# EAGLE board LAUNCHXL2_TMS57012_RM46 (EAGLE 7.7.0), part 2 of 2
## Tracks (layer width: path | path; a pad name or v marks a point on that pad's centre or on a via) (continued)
HERCULES_LIN1_TXD  (via drill 0.38 pad 0.69) (continued)
  Bottom 0.152: v58.09,41.15 58.09,58.61 57.65,59.04 51.78,59.04 51.48,59.35 51.48,63.18 51.17,63.48 48.28,63.48 47.98,63.79 47.98,66.09 47.68,66.4 25.12,66.4 J10.9 | v93.2,8.9 93.13,4.67 93.43,4.37 94.94,4.37 95.25,4.67 J6.4 | v85.56,28.32 85.56,28.11 85.27,27.81 85.26,23.32 84.95,23.01 78.35,23.01 78.04,22.71 78.08,14.22 76.76,12.75 76.45,12.39 v76.47,9.45 | v69.54,41.15 90.49,41.15 v90.75,40.9 91.21,40.43 91.21,40.39 v91.13,31.5
HERCULES_MR_PB  (via drill 0.38 pad 0.56, 0.38 pad 0.69)
  Top 0.152: S1.4 125.89,44.35 v119.43,44.35 117.94,44.35 S1.3 | v51.99,45.06 U7.40 | v119.43,49.92 120.14,49.92 120.14,51 U2.3 117.22,51 116.92,51.31 116.92,54.23 117.22,54.53 124.26,54.53 124.26,57.2 113.62,57.2 111.67,55.24 | 111.67,55.24 | 111.67,55.24 109.55,55.24 109.25,55.55 109.25,61.2 108.94,61.51 v95.87,61.51 | v79.48,51.61 52.56,51.46 v51.99,52.03 51.91,52.12 44.12,52.12 43.97,52.27 42.44,52.27 42.29,52.12 25.15,52.12 24.46,52.81 v17.68,52.81 | J1.15 4.83,53.21 4.65,53.03 v4.57,53.03 | v79.48,61.42 79.53,61.47 81.28,61.47 81.53,61.59 81.55,61.58 v92.56,61.58
  Bottom 0.152: v51.99,52.03 v51.99,45.06 | v119.43,44.35 v119.43,49.92 | v79.48,51.61 v79.48,61.42 | v4.57,53.03 4.57,52.5 7.01,50.06 15.32,50.06 16.38,51.36 17.53,52.81 v17.68,52.81 | v92.56,61.58 92.63,61.51 v95.87,61.51
HERCULES_NRST  (via drill 0.38 pad 0.69)
  Top 0.152: v56.16,57.81 55.52,57.78 53.47,57.78 53.09,58.04 34.92,58.04 34.59,57.81 34.29,57.51 J5.5 | v93.28,58.95 93.28,60.67 93.07,60.88 92.05,60.88 91.85,61.09 81.92,61.09 81.53,60.71 75.82,60.71 75.42,60.97 v74.73,61.54 | v57.51,62.91 v50.62,62.91 | v121.21,49.28 R10.1 | v54.93,35.26 U7.25 | v111.21,62.08 114.46,62.08 116.47,63.7 122.38,63.7 122.97,63.12 v123.29,63.12 | v97.79,62.08 v109.66,62.08 | J9.5 98.78,55.52 98.78,52.12 98.39,51.73 v92.71,51.73 | 124.39,33.31 | 124.39,33.31 S2.4 | S2.4 | 124.39,33.31 v123.05,33.31 S2.3
  Top 0.203: 99.59,47.92 99.16,47.57 98.88,47.57 98.81,47.3 98.81,46.79 | 98.81,46.79 98.81,45.34 | 98.81,46.79 v98.59,46.79
  Top 0.254: C3.1 99.59,47.92 | 98.81,45.34 U1.116
  Bottom 0.152: v93.28,58.95 96.24,58.95 96.55,58.65 96.55,56.52 J9.5 v97.79,62.08 | J10.22 57.15,63.82 v57.51,62.91 57.51,62.89 58.67,61.72 74.55,61.72 v74.73,61.54 | v123.05,33.31 123.05,45.25 121.21,47.09 v121.21,49.28 123.29,51.36 123.29,58.52 123.6,58.83 123.6,62.81 v123.29,63.12 | v50.62,62.91 50.62,58.91 50.93,58.61 55.28,58.61 v56.16,57.81 56.24,57.3 56.77,56.77 56.77,56.24 57,56.01 57,49.38 56.77,49.15 56.77,47.7 56.92,47.55 56.92,37.25 v54.93,35.26 | v109.66,62.08 v111.21,62.08 | v92.71,51.73 92.71,48.72 93.12,48.31 97.07,48.31 v98.59,46.79
HERCULES_NTRST  (via drill 0.38 pad 0.56, 0.38 pad 0.69)
  Top 0.152: v46.38,25.52 U7.107 | v68.82,48.88 68.81,48.9 68.2,48.9 68.07,48.77 52.32,48.77 51.96,49.14 v46.43,49.14 45.24,49.95 26.18,49.95 25.76,49.53 22.71,49.53 v22.55,49.76 | J1.2 v14.94,62.1 | v90.06,38.65 98.42,38.65 101.73,42.04 101.73,43.81 102.3,44.39 U1.109
  Bottom 0.152: v68.82,48.88 68.82,40.88 69.12,40.58 89.68,40.58 89.98,40.27 v90.06,38.65 | v46.43,49.14 45.09,47.67 45.09,40.46 46.38,39.17 v46.38,25.52 | v22.55,49.76 22.55,52.65 19.89,55.32 17.98,55.32 15.7,57.61 15.7,61.8 15.39,62.1 v14.94,62.1
HERCULES_RTCK  (via drill 0.38 pad 0.56, 0.38 pad 0.69)
  Top 0.152: v99.14,41.84 99.63,41.92 100.39,42.68 100.39,43.99 100.32,44.06 U1.113 | v86.48,38.17 87.1,37.87 87.4,37.57 v98.15,37.56 | v45.66,32.39 53.45,32.39 53.76,32.69 53.76,38.09 54.06,38.4 v67,38.4 | v46.25,22.87 46.49,22.87 46.79,23.16 U7.108 | J1.9 4.67,57.02 v4.72,56.92
  Bottom 0.152: v98.15,37.56 99.19,38.48 v99.14,41.84 | v67,38.4 74.61,38.4 74.85,38.16 81.7,38.16 83.46,39.92 86.19,39.92 86.33,39.78 86.33,38.79 86.49,38.71 86.49,38.56 v86.48,38.17 | v46.25,22.87 45.66,24.08 v45.66,32.39 44.56,31.3 44.56,29.55 44.26,29.25 41.66,29.25 41.27,29.63 41.27,40.13 41.02,40.39 41.02,41.4 41.27,41.66 41.27,45.09 40.64,45.72 36.2,45.72 35.69,46.23 21.19,46.19 20.88,46.49 20.88,53.73 20.04,54.57 15.3,54.57 15.01,55.02 15.01,56.08 14.71,56.39 5.11,56.39 v4.72,56.92
HERCULES_TCK  (via drill 0.38 pad 0.56, 0.38 pad 0.69)
  Top 0.152: v79.46,46.93 78.96,47.43 61.69,47.43 61.4,47.13 54.3,47.13 54,46.83 U7.35 | U1.112 100.8,42.35 99.47,41.02 98.65,41.02 98.15,41.67 v97.46,41.67 | v16,52.96 16.77,52.27 16.76,52.26 16.76,51.51 17.14,51.13 19.2,51.13 19.66,51.59 24.16,51.59 24.46,51.28 42.37,51.28 42.6,51.05 43.81,51.05 44.2,51.44 51.82,51.44 52.32,50.93 57.15,50.93 57.4,50.8 78.79,50.85 79.15,50.62 v79.46,50.09 | J1.11 7.02,55.7 4.57,55.7 v4.12,55.55
  Bottom 0.152: v97.46,41.67 97.46,42.72 96.77,43.41 96.77,44.45 95.89,45.34 79.99,45.34 79.46,45.88 v79.46,46.93 v79.46,50.09 | v4.12,55.55 8.53,55.55 9.98,54.1 14.55,54.1 v16,52.96
HERCULES_TDI  (via drill 0.38 pad 0.56, 0.38 pad 0.69)
  Top 0.152: v100.75,46.55 101.82,46.55 U1.110 | v52.59,42.66 52.78,42.47 | 52.78,42.47 | 52.78,42.47 U7.38 | 6.92,60.88 J1.3 6.94,60.81 5.03,60.81 2.59,58.37 2.59,50.9 4.19,49.3 14.33,49.3 15.28,50.25 21.68,50.25 22.1,50.67 23.32,50.67 23.7,50.29 49.3,50.29 49.76,49.84 52.35,49.84 v52.59,49.59 52.65,49.53 66.6,49.53 66.98,49.91 70.03,49.91 70.64,49.3 76.66,49.3 77.11,48.84 79.86,48.84 80.68,49.75 v80.95,49.75
  Bottom 0.152: v52.59,49.59 v52.59,42.66 | v100.75,46.55 100.69,46.18 81.99,46.18 80.47,47.7 80.47,48.77 80.92,49.23 80.92,49.72 v80.95,49.75
HERCULES_TDO  (via drill 0.38 pad 0.56, 0.38 pad 0.69)
  Top 0.152: v53.19,38.19 U7.37 | J1.7 4.04,58.29 v3.73,58.22 | v14.71,59.44 15.54,59.44 19.43,55.55 21.49,55.55 21.79,55.24 32.31,55.24 32.61,55.02 35.74,55.02 36.12,55.32 45.11,55.32 45.41,55.02 47.93,55.02 48.08,54.86 53.09,54.86 v53.03,54.89 | U1.111 101.35,45.28 101.35,44.32 101.22,44.07 101.22,42.16 99.43,40.38 98.2,39.27 88.77,39.27 87.55,40.39 84.67,40.38 84.37,40.81 84.37,44.14 83.81,45.46 55.21,45.46 55.02,45.26 55.02,44.61 v54.98,44.58
  Bottom 0.152: v53.19,38.19 53.11,41.83 53.26,42.14 53.26,42.67 53.19,43.05 53.19,45.42 | 53.19,45.42 53.11,48.92 53.34,49.23 53.34,49.84 53.11,50.14 v53.03,54.89 | v3.73,58.22 13.49,58.22 v14.71,59.44 | 53.19,45.42 54.15,45.42 v54.98,44.58
HERCULES_TMS  (via drill 0.38 pad 0.56, 0.38 pad 0.69)
  Top 0.152: v99.08,58.32 99.08,52.77 99.59,52.27 104.39,52.27 104.78,51.89 v104.78,51.56 | v54.57,54.89 55.12,54.86 | 55.12,54.86 54.99,54.86 | 55.12,54.86 74.42,54.86 74.55,54.99 75.31,54.99 75.44,54.86 80.26,54.86 80.77,54.48 84.71,54.48 85.18,54.59 85.41,55.12 85.41,55.99 v84.75,56.81 | v54.57,47.71 53.9,47.71 53.59,47.4 U7.36 | J1.1 v4.88,62.1 | v15.01,51.82 16.31,50.67 19.66,50.67 20.19,51.21 23.77,51.21 24.16,50.83 41.45,50.83 41.6,50.67 44.65,50.67 45.03,51.05 51.13,51.05 51.66,50.52 54.37,50.52 v54.5,50.32 | v104.78,48.22 104.78,44.58 104.27,44.07 104.27,43.35 U1.108
  Bottom 0.152: v84.75,56.81 84.75,63.93 85.05,64.24 88.16,64.24 89.59,62.73 98.78,62.73 99.08,62.34 v99.08,58.32 | v54.57,47.71 v54.5,50.32 v54.57,54.89 | v15.01,51.82 11.96,51.82 11.05,52.73 10.06,52.73 8.15,54.63 3.89,54.63 2.82,55.7 2.82,58.6 4.57,60.35 4.57,61.8 v4.88,62.1 | v104.78,48.22 104.78,49 105.16,49.38 105.16,49.99 104.85,50.29 104.85,51.48 v104.78,51.56
IRSTN  (via drill 0.38 pad 0.69)
  Top 0.152: R39.2 v38.12,34.41
  Top 0.178: R39.2 38.61,35.36 39.4,36.05 U7.70 | J12.10 v13.36,25.91
  Bottom 0.152: v38.12,34.41 39.5,34.42 40.51,33.53 40.51,28.07 39.88,27.43 37.72,25.4 37.72,25.38 37.34,25.15 35.05,25.15 34.82,25.38 34.59,25.38 27.18,25.4 26.04,25.02 20.07,25.02 19.18,25.91 v13.36,25.91
ITCK  (via drill 0.38 pad 0.69)
  Top 0.152: U7.100 43.59,25.65 44.15,26.21 v44.3,26.21 | 26.54,23.62 15.62,23.62 15.24,24 15.24,25.78
  Top 0.178: J12.4 14.73,29.72 15.24,29.21 15.24,25.78 | 26.54,23.62 29.59,19.56 38.73,19.56 v41.35,22.17
  Bottom 0.178: v41.35,22.17 41.35,23.27 v44.3,26.21
ITDI
  Top 0.152: 25.78,22.48 15.49,22.48 14.35,23.75 14.35,25.4
  Top 0.178: U7.98 42.8,21.84 39.5,18.41 28.7,18.41 25.78,22.48 | 14.35,25.4 14.35,26.8 14.1,27.05 11.3,27.05 J12.8
ITDO
  Top 0.152: U7.97 | 14.86,25.53 14.86,23.75 15.49,23.11 26.04,23.11
  Top 0.178: 42.37,24.21 U7.97 42.42,24.21 42.39,23.77 42.39,23.36 42.37,23.33 42.29,23.24 42.29,22.1 41.53,21.34 41.4,21.34 39.12,19.05 29.08,19.05 26.04,23.11 | J12.6 14.22,28.45 14.86,27.81 14.86,25.53
ITMS
  Top 0.152: 41.48,23.82 41.48,23.42 | 15.75,26.04 15.75,24.13 15.88,24 27.05,24
  Top 0.178: 41.48,23.82 41.48,24.84 41.99,25.35 43.08,25.35 43.18,25.25 U7.99 | J12.2 14.22,30.99 15.75,29.46 15.75,26.04 | 27.05,24 30.1,20.07 38.25,20.07 41.48,23.42
KGND
  Top 0.152: 82.8,34.39 U1.19
  Top 0.178: C2.2 C1.2 80.61,34.39 81.45,34.39 81.63,34.34 82.37,34.34 82.8,34.39
MIBSPI1CLK  (via drill 0.38 pad 0.69)
  Top 0.152: J6.7 101.6,12.06 101.6,14.86 101.91,15.16 102.37,15.16 102.67,15.47 102.67,27.75 102.37,28.05 100.28,28.05 99.98,28.36 v99.98,33.7 100.7,34.42 100.7,36.56 101,36.86 U1.95
  Bottom 0.152: v99.98,33.7 94.8,33.7 94.5,34.01 94.5,44.07 93.81,44.89 83.69,44.83 79.5,44.83 79.45,44.89 79.02,45.27 78.72,45.57 78.72,63.64 79.02,63.94 81.09,63.94 J10.32
MIBSPI1NCS_0/MIBSPI1SOMI_1/MII_TXD_2/ECAP6  (via drill 0.38 pad 0.56)
  Top 0.152: J9.3 92.71,59.77 92.28,60.2 91.82,60.2 91.31,60.71 82.42,60.71 81.92,60.2 71.37,60.2 68.96,62.61 68.96,63.75 J10.26 | U1.105 103.07,41.84 102.74,42.16 102.74,43.05 102.87,43.18 102.87,46.94 102.41,47.4 102.11,47.4 v101.58,47.85
  Bottom 0.152: J9.3 93.73,55.5 93.73,52.12 94.64,51.21 94.64,50.75 94.49,50.6 94.49,50.14 94.94,49.68 99.97,49.68 v101.58,47.85
MIBSPI1NCS_1/N2HET1_17/MII_COL/EQEP1S  (via drill 0.38 pad 0.69)
  Top 0.152: v90.73,47.73 90.89,47.54 91.81,46.61 U1.130 | v82.82,63.5 76.63,63.5 76.2,64.06 76.2,66.09 75.89,66.4 30.77,66.4 J10.11 | v82.82,60.1 90.51,60.1 v90.93,59.52 | v95,59.52 105.11,59.52 105.41,59.22 J9.8
  Bottom 0.152: v82.82,63.5 v82.82,60.1 82.83,58.22 82.37,57.76 82.37,56.39 82.82,55.94 82.82,55.64 82.83,55.63 82.82,48.77 83.12,48.34 84.75,48.34 84.96,48.13 85.98,48.13 86.23,48.39 90.19,48.39 v90.73,47.73 | v95,59.52 v90.93,59.52
MIBSPI1NCS_2/N2HET1_19/MDIO  (via drill 0.38 pad 0.69)
  Top 0.152: v86.33,25.15 86.33,25.87 86.49,26.04 87.16,26.04 v87.55,26.34 | v113.6,52.68 107.01,52.68 106.7,52.98 106.7,55.27 J9.9 | v86.33,25.15 | v86.33,25.15 U1.40
  Bottom 0.152: v86.33,25.15 86.33,22.44 86.02,22.14 81.31,22.14 81,21.83 81,2.9 J11.31 | v113.6,52.68 113.6,29.91 113.3,29.6 89.44,29.6 89.13,29.91 89.13,39.19 88.96,39.37 87.65,39.37 87.47,39.19 v87.55,26.34
MIBSPI1NENA/N2HET1_23/MII_RXD_2/ECAP4  (via drill 0.38 pad 0.69)
  Top 0.152: J8.4 93.85,55.37 v93.85,60.67 | v85.32,63.67 84.81,64.18 81.24,64.18 J10.31 | v100.13,37.28 103.73,37.28 103.8,37.34 U1.96
  Bottom 0.152: v85.32,63.67 85.32,60.97 85.62,60.67 v93.85,60.67 | J8.4 97.1,52.12 98.75,52.12 99.52,51.36 103.02,51.36 103.17,51.21 103.17,47.7 103.02,47.55 103.02,45.11 102.56,44.64 100.7,44.64 100.39,44.34 100.39,37.55 v100.13,37.28
MIBSPI1SIMO  (via drill 0.38 pad 0.69)
  Top 0.152: v110.5,38.47 110.5,36.15 110.2,35.84 U1.93 | J9.6 101.6,55.24 106.1,55.24 106.4,54.94 106.4,51.44 106.88,50.98 v110.48,50.98
  Bottom 0.152: J9.6 100.33,62.65 99.8,63.11 92.62,63.11 J10.35 | v110.48,50.98 110.48,50.93 v110.5,38.47
MIBSPI1SOMI  (via drill 0.38 pad 0.69)
  Top 0.152: v106.04,37.52 106.04,36.66 105.73,36.35 U1.94
  Bottom 0.152: J10.33 86.08,66.4 101.4,66.4 101.7,66.09 101.7,57.68 J9.7 101.7,55.35 101.7,53.56 102.11,52.96 105.46,52.96 105.77,52.65 105.77,52.19 105.77,52.18 105.77,43.69 106.08,43.38 106.28,43.38 106.58,43.08 106.58,42.52 105.47,41.4 105.47,38.09 v106.04,37.52
MIBSPI3CLK/AWM_EXT_SEL_1/EQEP1A  (via drill 0.38 pad 0.69)
  Top 0.152: v87.2,15.53 87.63,15.49 92.08,15.49 92.78,16.32 92.8,16.9 U1.53 | v87.24,6.77 v39.37,6.77 | v87.24,4.21 v97.79,4.21
  Bottom 0.152: 86.45,7.55 v87.24,6.77 v87.24,4.21 | 86.45,7.55 | 86.45,7.55 86.45,14.94 v87.2,15.53 | v39.37,6.77 J2.7 | v97.79,4.21 J11.38
MIBSPI3NCS_0/AD2EVT/GIOB_2/EQEP1I  (via drill 0.38 pad 0.69)
  Top 0.152: v93.14,25.26 93.82,25.26 U1.55 | J6.5 97.79,9.63 98.09,9.32 111.73,9.32 112.03,9.63 112.03,26.77 v112.09,26.9 112.62,26.83 113.54,25.91 | 123.12,23.15 S3.3 113.76,23.15 113.54,23.37 113.54,25.91 | 123.12,23.15 | 123.12,23.15 S3.4 | S3.4 | 113.54,25.91 113.79,26.16 R13.1
  Bottom 0.152: J6.5 97.79,5.84 98.09,5.54 102.56,5.54 102.87,5.23 J11.40 | v112.09,26.9 112.03,26.89 100.13,26.82 99.9,27.28 97.69,27.28 96.32,28.65 94.72,28.65 94.34,28.04 94.34,27.77 93.14,26.58 v93.14,25.26
MIBSPI3NCS_1/N2HET1_25/MDCLK  (via drill 0.38 pad 0.69)
  Top 0.152: v64.99,58.08 64.99,59.49 63.92,60.3 38.89,60.3 v37.53,61.4 | v37.53,61.4 | v77.47,21.12 69.56,21.12 69.25,21.43 69.25,26.79 70.97,28.5 70.97,34.11 v72.95,35.94 | v84.69,25.42 84.83,25.28 U1.37
  Bottom 0.152: v37.53,61.4 33.35,61.4 33.05,61.1 33.05,52.98 32.74,52.68 30.95,52.68 30.64,52.98 30.64,55.08 J5.3 | v72.95,35.94 65.29,35.94 64.99,36.25 v64.99,58.08 | v84.69,25.42 82.82,23.55 77.78,23.55 77.47,23.25 v77.47,21.12 77.47,14.43 75.89,12.8 75.69,12.6 75.74,4.95 75.44,4.65 75.44,3.73 75.69,3.48 75.69,3.15 J11.30
MIBSPI3NCS_2/I2C_SDA/N2HET1_27/NTZ2  (via drill 0.38 pad 0.69)
  Top 0.152: v62.46,42.68 63.36,43.2 69.85,43.18 70.1,43.18 | 78.42,41.84 78.49,41.84 | 78.49,41.84 U1.4 | v56.02,50.17 v62.46,50.17 | v22.23,15.24 24.26,15.24 24.77,15.75 25.43,16.42 25.73,16.73 66.63,16.73 66.93,17.03 66.93,32.69 70.19,35.87 70.18,37.87 70.79,38.56 70.79,42.22 70.11,42.73 70.1,43.18 | 70.1,43.18 77.11,43.18 78.3,41.86 78.46,41.86 78.49,41.84
  Bottom 0.152: v62.46,50.17 v62.46,42.68 | v56.02,50.17 56.02,50.2 55.4,50.83 55.41,56.74 54.62,57.53 48.64,57.53 48.26,57.91 44.07,57.91 42.67,56.52 J5.8 | v22.23,15.24 21.72,14.61 21.72,10.79 24,8.64 24,2.92 J11.9
MIBSPI3NCS_3/I2C_SCL/N2HET1_29/NTZ1  (via drill 0.38 pad 0.69)
  Top 0.152: v59.62,43.76 77.45,43.76 78.86,42.35 U1.3 | J5.9 45.7,55.42 52.1,55.42 52.37,55.54 v59.62,55.54 | v43.18,51.69 24.74,51.69 24.31,52.12 19.18,52.12 v18.82,51.84
  Bottom 0.152: J5.9 43.18,55.24 v43.18,51.69 | J11.8 20.4,0.71 18.09,0.71 17.78,1.02 17.78,2.34 14.48,5.64 14.48,7.16 13.87,7.77 13.44,7.77 13.36,7.86 3.7,7.86 3.4,8.16 3.4,27.48 4.04,28.12 4.19,28.32 4.19,31.11 3.3,32.13 1.91,33.27 1.91,48.9 2.79,49.78 5.97,49.78 6.22,49.53 16.51,49.53 v18.82,51.84 | v59.62,55.54 v59.62,43.76
MIBSPI3NENA/MIBSPI3NCS_5/N2HET1_31/EQEP1B  (via drill 0.38 pad 0.69)
  Top 0.152: v99.13,17.95 98.86,17.68 97.61,17.68 97.54,17.6 93.73,17.6 93.62,17.72 93.31,18.02 U1.54 | v100.33,6.66 v100.33,4.97
  Bottom 0.152: J6.8 105.41,6.97 105.11,6.66 v100.33,6.66 100.33,7.27 99.13,8.47 v99.13,17.95 | v100.33,4.97 J11.39
MIBSPI3SIMO/AWM_EXT_SEL_0/ECAP3  (via drill 0.38 pad 0.69)
  Top 0.152: v89.19,8.88 v60.93,8.88 | v60.93,23.6 55.44,23.6 55.13,23.9 55.13,26.14 51.43,29.84 v43.24,29.84 | v89.19,16.41 92.02,16.41 92.32,16.84 U1.52
  Bottom 0.152: J11.37 94.06,0.71 91.75,0.71 91.44,1.02 91.44,4.07 89.19,6.32 v89.19,8.88 89.18,8.9 89.18,15.76 v89.19,16.41 | v43.24,29.84 43.24,49.16 42.94,49.47 35.89,49.47 35.59,49.77 35.59,55.27 J5.6 | v60.93,23.6 v60.93,8.88
MIBSPI3SOMI/AWM_EXT_ENA/ECAP2  (via drill 0.38 pad 0.69)
  Top 0.152: v56.17,40.27 v67.79,40.27 | v91.47,17.72 91.94,18.19 91.94,22.55 91.81,22.67 U1.51
  Bottom 0.152: v91.47,17.72 | v91.47,17.72 91.47,9.13 92.71,7.89 J11.36 | v91.47,17.72 89.22,17.72 88.93,18.01 | 88.93,18.01 | 88.93,18.01 81.85,18.01 81.55,18.32 81.55,21.26 81.85,21.57 86.59,21.57 86.94,21.92 86.94,25.38 86.87,34.29 86.87,35.36 87.17,35.59 87.1,39.85 86.59,40.27 v67.79,40.27 | v56.17,40.27 56.16,49.38 56.17,49.38 56.17,49.46 56.62,49.91 56.62,50.67 56.16,51.13 56.17,56.67 54.67,58.17 49.66,58.17 49.28,58.55 41.4,58.55 J5.7
MIBSPI5CLK/MII_TXEN/RMII_TXEN  (via drill 0.38 pad 0.69)
  Top 0.152: J8.10 109.25,53.98 108.94,54.28 108.94,60.36 108.64,60.67 95.03,60.67 94.73,60.97 94.73,62.19 94.42,62.5 75.51,62.56 75.36,62.71 74.14,62.71 73.93,62.5 72.76,62.5 J10.27 | v108.83,38.8 106.42,38.8 105.87,39.35 U1.100
  Bottom 0.152: J8.10 110.49,52.18 108.83,50.52 | 108.83,50.52 | 108.83,50.52 v108.83,38.8
MIBSPI5NCS_0/EPWM4A  (via drill 0.38 pad 0.69)
  Top 0.152: U1.32 82.91,27.81 84.05,27.81 84.12,27.74 84.12,27.19 v84.15,27.16
  Bottom 0.152: v84.15,27.16 81.35,25.12 78.39,25.12 78.12,25.39 67.61,25.39 67.31,25.08 J11.26
MIBSPI5NENA/MII_RXD_3/MIBSPI5SOMI_1/ECAP5  (via drill 0.38 pad 0.69)
  Top 0.152: v87.06,63.59 86.33,64.01 86.33,66.06 86.07,66.4 78.46,66.4 J10.30 | J8.5 96.55,55.22 96.55,57.73 v97.12,58.31 | v103.05,37.85 U1.97
  Bottom 0.152: v97.12,58.31 97.12,61.77 96.74,62.23 87.44,62.23 87.06,62.53 v87.06,63.59 | v103.05,37.85 103.33,38.13 103.33,47.09 103.33,47.4 103.48,47.55 103.48,51.51 103.33,51.66 101.35,51.66 100.74,52.27 99.49,52.27 J8.5
MIBSPI5SIMO_0/MII_TXD_1/RMII_TXD_1/MIBSPI5SOMI_2  (via drill 0.38 pad 0.56, 0.38 pad 0.69)
  Top 0.152: v101.38,38.46 102.32,38.46 102.72,38.86 104.09,38.86 U1.99 | J9.4 95.25,57.74 94.42,58.57 94.42,61.81 94.06,62.18 91.75,62.18 91.59,62.03 80.92,62.03 80.77,62.18 78.94,62.18 78.49,61.72 75.74,61.72 75.29,62.26 74.22,62.26 73.98,62.12 71.49,62.12 v70.1,63.5
  Bottom 0.152: J9.4 95.25,55.27 95.56,54.97 98.77,54.97 99.07,54.66 99.07,53.18 99.52,52.73 100.89,52.73 101.35,52.27 103.63,52.27 103.94,51.97 103.94,50.29 103.78,49.99 103.78,47.55 103.94,47.4 103.94,37.58 103.33,36.98 102.6,36.98 101.38,37.43 v101.38,38.46 | v70.1,63.5 71.88,63.5 72.14,63.75 72.14,65.15 J10.28
MIBSPI5SOMI_0/MII_TXD_0/RMII_TXD_0  (via drill 0.38 pad 0.69)
  Top 0.152: J9.10 110.49,62.5 110.12,62.87 95.25,62.87 95,63.12 88.21,63.12 88.01,62.99 84.96,62.99 84.84,63.12 83.44,63.12 83.19,62.87 82.42,62.87 82.3,62.99 75.56,62.99 75.36,63.18 74.93,63.49 J10.29 | U1.98 107.49,38.36 108.66,37.19 109.41,37.19 v109.51,37.29
  Bottom 0.152: J9.10 111.56,55.45 111.56,53.34 111.25,53.03 111.25,50.75 111.1,50.6 111.1,39.47 111.48,39.09 111.48,38.33 110.8,37.64 109.86,37.64 v109.51,37.29
N2HET1_0/SPI4CLK/EPWM2B  (via drill 0.38 pad 0.69)
  Top 0.152: v84.08,31.35 U1.25
  Bottom 0.152: v84.08,31.35 80.24,31.35 78.83,29.93 60.58,29.93 60.27,29.63 60.27,4.66 59.97,4.36 54.52,4.36 J11.20
N2HET1_1/SPI4NENA/N2HET2_8/EQEP2A  (via drill 0.38 pad 0.69)
  Top 0.152: v77.91,58.95 v87.96,58.95 | v93.69,32.34 93.34,32.51 85.17,32.51 v85.09,32.59 84.84,32.34 U1.23 | U1.23
  Bottom 0.152: J11.21 56.41,3.7 61.42,3.7 61.73,4.01 61.73,29.22 62.03,29.53 73.94,29.53 74.94,28.52 79.51,28.52 80.3,29.31 84.34,29.31 84.8,29.62 84.8,31.36 85.09,31.8 v85.09,32.59 | v93.69,32.34 93.69,43.64 93.13,44.45 83.69,44.45 79.63,44.45 79.24,44.45 78.47,45.09 77.91,45.65 v77.91,58.95 | v87.96,58.95 90.17,56.74 J9.2
N2HET1_2/SPI4SIMO/EPWM3A  (via drill 0.38 pad 0.69)
  Top 0.152: v84.08,28.74 83.96,28.86 U1.30
  Bottom 0.152: v84.08,28.74 83.89,28.92 81.09,28.92 80.12,27.95 62.53,27.95 62.23,27.65 J11.24
N2HET1_3/SPI4NCS_0/N2HET2_10/EQEP2B  (via drill 0.38 pad 0.69)
  Top 0.152: v71.12,24.82 77.51,24.82 77.81,25.12 77.81,31.55 78.12,31.86 U1.24
  Bottom 0.152: v71.12,24.82 71.12,1.02 70.81,0.71 58.34,0.71 J11.22
N2HET1_4/EPWM4B  (via drill 0.38 pad 0.69)
  Top 0.152: v69.85,9.45 45.79,9.45 J2.9 | v69.85,23.68 82.54,23.68 82.85,23.98 U1.36
  Bottom 0.152: J11.27 v69.85,9.45 v69.85,23.68
N2HET1_5/SPI4SOMI/N2HET2_12/EPWM3B  (via drill 0.38 pad 0.69)
  Top 0.152: v81.36,28.35 U1.31
  Bottom 0.152: v81.36,28.35 81.36,26.99 81.06,26.68 65.08,26.68 64.77,26.38 J11.25
N2HET1_6/SCIRX/EPWM5A  (via drill 0.38 pad 0.69)
  Top 0.152: J11.33 81.62,5.38 49.48,5.38 49.02,5.89 45.36,5.89 44.86,5.49 33.56,5.49 29.21,9.54 J2.3 | v85.08,17.07 85.08,17.42 85.34,17.68 U1.38
  Bottom 0.152: J11.33 85.09,16.85 v85.08,17.07
N2HET1_7/N2HET2_14/EPWM7B  (via drill 0.38 pad 0.69)
  Top 0.152: v72.54,24.25 78.43,24.25 78.73,24.55 78.73,27.22 79.03,27.53 81.6,27.53 81.77,27.36 U1.33
  Bottom 0.152: v72.54,24.25 J11.28
N2HET1_8/MIBSPI1SIMO_1/MII_TXD_3  (via drill 0.38 pad 0.69)
  Top 0.152: J8.3 91.16,55.52 91.16,57.51 90.86,57.81 v86.22,57.81 71.26,57.81 66.34,62.73 | 66.34,62.73 | 66.34,62.73 v62.23,62.73 | v106.82,45.53 105.81,45.53 105.35,45 105.35,44.04 105.25,43.94 105.25,42.35 U1.106 | v96.44,60.1 v106.13,60.1
  Bottom 0.152: v62.23,62.73 J10.24 | v106.13,60.1 106.4,59.83 106.4,55.3 106.91,54.63 106.91,53.42 107.44,52.88 107.44,46.15 v106.82,45.53 | v96.44,60.1 89.08,60.1 88.72,59.74 86.64,59.74 86.22,59.32 v86.22,57.81
N2HET1_9/N2HET2_16/EPWM7A  (via drill 0.38 pad 0.69)
  Top 0.152: v74.93,10.79 J2.10 | v81.61,24.34 81.61,26.34 U1.35
  Bottom 0.152: v81.61,24.34 75.23,24.34 74.93,24.03 v74.93,10.79 J11.29
N2HET1_10/MII_TX_CLK/MII_TX_AVCLK4/NTZ3  (via drill 0.38 pad 0.69)
  Top 0.152: v58.82,53.75 79.04,53.75 79.26,53.98 v80.23,53.98 86.33,53.98 | 86.33,53.98 | 86.33,53.98 J8.1 | J8.1 | v97.46,43.83 97.81,44.17 U1.118
  Bottom 0.152: v58.82,53.75 58.82,59.11 58.39,59.54 52.38,59.54 52.07,59.84 J10.20 | v80.23,53.98 80.26,49.15 80.01,48.9 80.01,47.88 80.19,47.55 80.19,46.69 81.15,45.72 97.03,45.72 97.46,45.29 v97.46,43.83
N2HET1_11/MIBSPI3NCS_4/N2HET2_18/EPWM1SYNCO  (via drill 0.38 pad 0.56, 0.38 pad 0.69)
  Top 0.152: v72.46,58.65 72.73,58.38 v91.88,58.38 | v79.39,39.7 81.07,40.85 U1.6 | v63.5,39.62 v66.04,39.62
  Bottom 0.152: J11.11 30.48,3.17 30.48,15.81 30.79,16.12 53.15,16.12 53.45,16.42 53.45,34.21 53.76,34.52 57.49,34.52 62.46,39.62 v63.5,39.62 | v91.88,58.38 95.94,58.38 96.24,58.08 96.24,55.58 96.55,55.27 100.03,55.27 100.33,54.97 J8.6 | v72.46,58.65 70.89,58.65 67.22,54.98 | 67.22,54.98 | 67.22,54.98 67.21,41.3 67.21,40.79 v66.04,39.62 67.45,39.62 67.52,39.7 v79.39,39.7
N2HET1_12/MII_CRS/RMII_CRS_DV  (via drill 0.38 pad 0.69)
  Top 0.152: v92.89,43.22 94.25,43.22 94.63,43.53 94.63,43.78 94.81,43.96 U1.124 | v56.53,60.97 56.48,61.02 46.61,61.02 v46.48,60.9
  Bottom 0.152: 45.22,59.63 v46.48,60.9 46.48,64.9 J10.18 | 45.22,59.63 | 45.22,59.63 38.41,59.63 38.1,59.33 38.1,55.24 J4.6 | v56.53,60.97 56.54,60.96 58.04,60.96 75.63,60.97 75.93,60.67 75.93,44.46 76.33,44.07 78.36,44.07 78.49,44.2 78.99,44.2 79.12,44.07 79.76,44.07 80.01,43.81 88.77,43.81 89.03,44.07 89.66,44.07 89.92,43.81 92.14,43.81 v92.89,43.22
N2HET1_13/SCITX/EPWM5B  (via drill 0.38 pad 0.69)
  Top 0.152: J2.4 33.02,12.06 35.26,12.06 35.56,12.37 35.56,14.19 35.87,14.5 39.8,14.5 40.29,14.99 49.53,14.99 50.8,13.72 76.71,13.72 77.98,15.11 85.22,15.11 v85.73,15.58 86.15,15.98 86.15,16.44 85.88,16.71 85.88,22.79 85.89,22.79 85.83,22.89 85.81,23.21 85.88,23.88 U1.39
  Bottom 0.152: v85.73,15.58 86.08,15 86.08,3.45 J11.34
N2HET1_14  (via drill 0.38 pad 0.69)
  Top 0.152: U1.125 94.33,44.14 94.02,43.83 92.47,43.83 92.08,43.43 92.08,42.45 v91.86,42.05 | J10.17 45.71,64.15 v48.64,64.15
  Bottom 0.152: J10.17 39.43,60.38 35.59,60.38 35.28,60.08 35.28,54.97 J4.5 | v48.64,64.15 50.49,64.15 50.8,64.45 50.8,66.09 51.1,66.4 53.03,66.4 53.34,66.09 53.34,60.21 53.65,59.91 73.04,59.91 73.34,59.6 73.34,41.76 73.64,41.45 89.77,41.45 90.04,41.66 90.04,42.8 90.3,43.18 91.57,43.18 v91.86,42.05
N2HET1_15/MIBSPI1NCS_4/ECAP1  (via drill 0.38 pad 0.69)
  Top 0.152: J11.35 91.16,2.9 114,2.9 114.3,2.59 114.3,1.02 114.61,0.71 129.74,0.71 130.04,1.02 130.04,12.69 129.74,12.99 S4.4 | v86.54,17.28 86.54,22.48 86.81,22.75 U1.41 | S4.4 | S4.4 124.59,12.99 | 124.59,12.99 | 124.59,12.99 S4.3 117.78,12.83 114.68,12.83 114.41,13.1 R17.1
  Bottom 0.152: J11.35 88.62,3.45 88.62,15.2 v86.54,17.28
N2HET1_16/EPWM1SYNCI/EPWM1SYNCO  (via drill 0.38 pad 0.69)
  Top 0.152: v61.96,53.17 62.23,52.91 85.79,52.91 86.61,51.97 86.61,50.8 86.61,48.27 86.61,46.99 87.32,46.29 U1.139 | v61.96,57.62 60.78,57.62 59.63,58.46 24.99,58.45 24.54,58.83 24.54,63.09 23.93,63.7 20.75,63.7 J10.7
  Bottom 0.152: J4.3 29.21,54.97 28.91,55.27 28.25,55.27 27.94,55.58 27.94,62.09 27.64,62.4 23.56,62.4 22.25,63.7 20.75,63.7 J10.7 | v61.96,57.62 v61.96,53.17
N2HET1_18/EPWM6A
  Top 0.152: J4.2 28.04,52.6 45.09,52.58 51.18,52.58 51.44,52.7 52.58,52.7 53.34,52.07 85.61,52.22 85.79,52.05 85.98,51.82 86.23,51.44 86.23,46.86 86.81,46.23 U1.140
  Bottom 0.152: J4.2 25.39,55.33 22.85,55.33 21.41,56.77 19.2,56.77 17.07,58.9 17.07,64.85 J10.6
N2HET1_20/EPWM6B  (via drill 0.38 pad 0.69)
  Top 0.152: v40.84,46.94 50.33,46.94 51.67,48.28 79.4,48.28 80.04,47.6 80.22,47.55 83.69,47.55 83.82,47.88 85.09,47.88 85.6,47.12 85.6,46.86 86.33,46.13 U1.141
  Bottom 0.152: J10.5 16.34,62.34 16.34,57.7 17.87,56.17 20,56.17 21.97,53.98 J4.1 24.13,47.24 24.43,46.94 35.69,46.99 36.32,46.35 40.26,46.35 v40.84,46.94
N2HET1_22  (via drill 0.38 pad 0.69)
  Top 0.152: v42.41,30.43 v54.93,30.43 | v84.08,36.42 84.02,36.35 U1.15 | v56.41,23.02 v59.09,23.02
  Bottom 0.152: J11.17 43.18,3.17 43.18,14.08 43.81,14.61 43.94,14.73 50.93,14.73 51.69,13.97 55.24,13.97 56.11,14.76 56.41,15.07 v56.41,23.02 56.41,28.94 v54.93,30.43 | J5.2 26.67,55.49 27.1,55.49 27.94,54.65 27.94,48.06 28.25,47.62 34.34,47.62 35.46,49.02 41.27,49.02 41.78,47.88 41.78,41.27 41.53,41.02 41.53,40.51 41.78,40.26 41.78,31.05 v42.41,30.43 | v59.09,23.02 59.36,23.29 59.36,32.68 59.66,32.98 64.17,32.98 64.48,33.29 64.48,34.08 64.78,34.39 83.77,34.39 84.08,34.69 v84.08,36.42
N2HET1_24/MIBSPI1NCS_5/MII_RXD_0/RMII_RXD_0  (via drill 0.38 pad 0.69)
  Top 0.152: J6.9 109.25,12.09 109.25,19.19 111.14,21.09 111.14,33.41 v110.16,34.93 107.25,34.93 107.17,34.85 U1.91 | v108.94,63.68 v98.36,63.68
  Bottom 0.152: v98.36,63.68 96.98,63.68 J10.37 | v110.16,34.93 108.25,36.3 108.25,52.47 108.94,53.15 v108.94,63.68
N2HET1_26/MII_RXD_1/RMII_RXD_1  (via drill 0.38 pad 0.69)
  Top 0.152: 111.48,35.06 111.48,11.79 J6.10 | 111.48,35.06 111.04,35.5 105.83,35.5 105.69,35.36 U1.92 | 111.48,35.06 111.78,35.37 v115.33,35.37 | v119.37,65.82 118.8,66.4 93.7,66.4 J10.36
  Bottom 0.152: v119.37,65.82 119.37,64.36 117.2,62.19 117.2,50.92 117.79,50.33 117.79,49.01 117.48,48.71 115.51,48.71 115.21,48.4 v115.33,35.37
N2HET1_28/MII_RXCLK/RMII_REFCLK/MII_RX_AVCLK4  (via drill 0.38 pad 0.56)
  Top 0.152: U1.107 103.32,42.85 103.25,42.93 103.25,47.24 102.72,47.78 102.72,48.92 102.41,49.23 v102.18,49.23
  Bottom 0.152: J10.23 60.68,66.4 83.66,66.4 83.96,66.09 83.96,54.89 84.28,54.63 84.35,54.56 85.5,54.56 85.83,54.74 85.93,54.97 86.03,55.02 89.26,55.04 J8.2 90.22,53.92 90.22,51.66 90.37,51.51 91.75,51.51 91.9,51.66 91.9,52.12 92.35,52.58 93.12,52.58 93.42,52.27 93.42,51.82 93.57,51.66 93.57,49.23 93.88,48.92 99.67,48.92 101.35,47.24 102.26,47.24 102.41,47.4 102.41,49 v102.18,49.23
N2HET1_30/MII_RX_DV/EQEP2S  (via drill 0.38 pad 0.69)
  Top 0.152: v91.58,50.67 93.01,50.67 93.31,50.37 U1.127 | J10.14 40.08,62.16 65.38,62.16 69.78,57.89 70.61,57.28 82.53,57.3 82.65,57.43 85.39,57.43 85.98,56.77 85.98,55.24 86.11,55.12 88.52,55.12 89.03,54.61 89.03,53.09 89.28,52.83 v89.29,52.22
  Bottom 0.152: J10.14 33.48,62.05 33.05,62.05 32.74,61.75 32.74,54.97 J4.4 | v91.58,50.67 90.61,50.67 89.29,51.98 v89.29,52.22
N$1
  Top 0.152: U7.4 57.48,26.85 57.96,27.33 63.81,27.33 R32.1
N$2
  Top 0.152: R32.2 LED7.A
N$3
  pour Route15 (no thermals): 17.4,11.81 17.4,9.97 25.02,9.97 25.02,11.81
N$4
  pour Route15 (no thermals): 17.21,14.61 17.14,12.45 25.21,12.45 25.21,14.61
N$5
  pour Route15 (no thermals): 81.6,11.87 81.6,9.78 88.58,9.78 88.58,9.84 88.77,9.84 88.77,11.87
N$6
  Top 0.152: U7.3 56.23,26.44 57.72,26.44 58.06,26.77 62.53,26.77 63.2,26.11 R33.1
N$7
  Top 0.152: R45.2 26.14,20.17 25.65,19.68 23.75,19.68 23.75,19.19 R43.1
  Top 0.381: U9.5 21.21,19.02 C54.1 23.57,19.02 R43.1
N$8
  Top 0.152: R42.2 24.64,19.01 24.64,17.4 24.26,17.02 20.6,17.02 20.02,16.48 19.33,15.85 15.49,15.85 14.76,15.19 14.76,14.12 14.73,11.18 14.73,7.87 15.14,7.42 15.13,6.95 15.13,6.9 14.78,6.55 14.24,6.55 LED9.A
N$9
  Top 0.305: L1.2 21.6,31.24 22.72,31.24 23.01,31.45 23.01,33.58 23.2,33.77 U5.5
N$11
  Top 0.152: U5.8 25.15,34.49 25.15,33.58 25.59,32.93 R19.1 R18.1
N$12
  Top 0.305: L2.1 21.43,43.69 22.86,43.69 23.2,43.34 U5.16
N$13
  Top 0.152: R21.2 18.84,35.15 19.66,35.15 20.31,34.5 U5.1
  Top 0.305: R21.2 C28.1
N$14
  pour Route15 (no thermals): 81.53,14.35 81.53,12.45 88.96,12.45 88.84,14.29
N$16
  Top 0.152: LED6.A 17.4,26.29 16.64,27.05 16.64,30.86 15.62,31.88 15.62,32.46 R27.1
N$17
  Top 0.152: U5.13 25.2,40.23 25.2,41.2 25.77,41.63 R26.2 R25.2
N$21
  Top 0.152: R22.1 42.91,42.53 43.18,42.8 44.2,42.8 44.2,43.32 LED4.A
N$23
  Top 0.381: C52.1 R41.2 14.35,17.55 14.91,17.09 17.2,17.09 17.75,17.45 U9.3
N$33
  Top 0.152: U2.4 122.22,51 122.22,50.55 R9.1 R8.2
N$34
  Top 0.152: LED1.C 124.98,55.34 R11.2
N$35
  Top 0.152: R16.1 115.84,17.93 LED3.C
N$36
  Top 0.152: R15.1 116.5,24.04 116.84,24.38 117.86,24.38 118.62,25.15 118.62,26.04 119.13,26.54 119.13,28.7 118.87,28.96 116.7,28.96 LED2.C
N$39
  Top 0.152: R5.2 80.91,27.06 81.12,26.85 U1.34
N$41
  Top 0.254: R28.2 35.74,39.06 35.31,39.5 35.31,42.29 36.96,43.94 36.96,46.23 37.08,46.35 U6.6
N$43
  Top 0.152: R30.2 58.29,25.67 U7.1
N$58
  Top 0.152: R33.2 LED8.A
N$59
  Top 0.178: R31.2 54.3,22.55 54,22.91 U7.126
NERROR  (via drill 0.38 pad 0.69)
  Top 0.152: v85.32,42.05 85.72,41.45 86.94,41.45 87.62,40.92 89.06,39.7 95.99,39.7 96.65,40.51 96.65,41.91 97.16,42.42 97.92,42.42 98.3,42.8 98.3,43.74 v98.64,44.09 98.64,44.12 98.34,44.43 98.34,45.32 U1.117 | R11.1 116.16,56.52 115.85,56.21 115.85,50.62 115.55,50.32 103.33,50.29 103,50.73 v102.28,50.73
  Bottom 0.152: v85.32,42.05 84.81,42.37 74.27,42.35 73.97,42.66 73.97,59.91 73.54,60.47 57.4,60.45 57.28,60.45 57.15,60.33 56.26,60.33 56.13,60.45 55.05,60.45 55.04,60.47 54.61,61.02 J10.21 | v98.64,44.09 99.71,45.16 101.67,45.16 102.72,46.21 102.72,47.7 102.79,47.78 102.79,49.53 102.28,50.05 v102.28,50.73
NPORRST  (via drill 0.38 pad 0.69)
  Top 0.152: 120.29,52.88 | 120.29,52.88 | 120.29,52.88 120.29,51.94 U2.5 | R7.1 123.05,53.92 122.74,54.23 120.87,54.23 v120.29,53.66 120.29,52.88 | v89.7,25.11 89.67,25.11 89.32,24.77 U1.46 | 120.29,52.88 U2.1
  Bottom 0.152: v120.29,53.66 120.29,27.7 119.99,27.4 112.5,27.4 112.39,27.51 111.71,27.51 111.63,27.43 110.57,27.43 110.41,27.28 100.58,27.28 98.68,29.18 94.51,29.18 92.57,27.09 92.57,25.42 92.14,24.99 91.95,24.77 90.68,24.77 90.33,25.11 v89.7,25.11
OSC0
  Top 0.152: U7.88 38.1,28.86 | 38.1,28.86 33.68,28.86 32.51,30.02 32.51,32.56 32.41,32.66 32.41,33.38 Y2.2 | C34.1 38.09,28.92 38.1,28.86
OSC1
  Top 0.152: U7.89 38.1,28.45 | 38.1,28.45 38.1,28.25 38.1,27.75 C39.1 | 38.1,28.45 33.53,28.45 32.56,27.48 32.56,23.88 Y2.1
OSCIN
  Top 0.152: JP1.1 74.35,37.3 74.73,36.93 75.59,36.93 75.61,38.35 Y1.2 75.64,36.88
  Top 0.178: 75.61,38.35 75.61,34.29 C1.1 79.5,34.38 79.5,34.95 81.18,34.95 81.28,34.85 U1.18
OSCOUT
  Top 0.152: 75.48,30.75 Y1.1 75.59,30.77 | U1.20
  Top 0.178: 75.59,30.77 75.59,33.27 C2.1 79.41,32.71 79.45,32.61 81.18,32.61 81.38,32.87 81.38,33.68 81.52,33.84 81.76,33.84 82.57,33.84 82.8,33.88 U1.20
USB_HIPWR_ENA  (via drill 0.38 pad 0.69)
  Top 0.152: v44.99,22.06 44.97,21.91 44.97,18.22 44.41,17.79 26.66,17.79 26.16,18.29 26.16,19.01 R45.1 | v50.08,25.75 50.69,25.67 50.8,25.18 U7.118
  Bottom 0.152: v50.08,25.75 50.14,25.68 50.22,24 50.23,21.56 49.85,21.18 46.02,21.18 v44.99,22.06
USB_ID  (via drill 0.38 pad 0.69)
  Top 0.178: U7.95 39.27,26.06 38.76,25.6 37.69,24.54 37.69,22.33 36.07,20.57 30.48,20.57 27.3,24.51 18.97,24.51 v18.49,25.25
  Top 0.305: J13.4 5.52,17.77 v5.54,17.78 | U10.4 8.79,17.96 v8.79,16.51
  Bottom 0.152: PAD14.1 7.85,16.66 | v5.54,17.78 J13.4 3.98,18.09 3.98,24.55 4.45,25.02 12.95,25.02 13.42,25.23 15.69,25.23 v18.49,25.25
  Bottom 0.305: PAD14.1 6.88,17.17 v5.54,17.78 | 7.85,16.66 v8.79,16.51
USB_PWRFAULT
  Top 0.152: LED9.C 12.8,6.58 12.8,7.32 14.22,8.26 14.22,15.54 14.99,16.28 18.64,16.28 20.07,17.4 20.07,17.91 U9.4
USB_SHIELD
  Top 0.356: J13.S4 1.57,14.66 1.57,12.9 1.94,12.54 C53.2 1.94,12.4 2.34,12.8 4.27,12.8 4.47,12.6 4.47,12.11 R44.1 | J13.S4 1.96,14.71 2.79,15.54 3.9,15.54 J13.S2 | J13.S4 1.68,14.77 1.68,15.7 1.63,15.75 J13.S6 J13.S5 1.63,21.34 2.16,21.87 | J13.S3 1.91,22.11 2.16,21.87 | 2.16,21.87 2.69,21.34 3.85,21.34 J13.S1
USBD_N  (via drill 0.38)
  Top 0.178: U7.93 42.4,26.85 v42.9,27.43
  Top 0.305: U10.1 6.25,18.97 v6.25,19.2
  Top 0.356: J13.2 5.38,19.09 6.1,19.09 6.15,19.14 6.2,19.14 v6.25,19.2
  Bottom 0.356: 42.62,27.01 42.61,27.01 arc90 v42.9,27.43 arc-90 42.58,27.04 42.24,27.04 arc90 40.65,25.48 arc-90 39.62,24.42 25.4,24.42 arc90 21.93,20.95 21.93,20.32 arc-90 20.95,19.34 19.05,19.34 arc-90 18.71,19.68 arc90 16.51,21.88 9.53,21.88 arc90 8.34,20.7 8.34,19.61 arc-90 7.77,19.04 6.41,19.04 v6.25,19.2 5.61,20.04 5.61,20.7 PAD16.1
USBD_P  (via drill 0.38)
  Top 0.178: U7.94 42.39,26.45 v42.67,25.93
  Top 0.305: U10.2 6.25,18.47
  Top 0.356: J13.3 5.13,18.41 5.31,18.52 5.89,18.5 6.07,18.4 v6.25,18.29 6.25,18.47
  Bottom 0.356: 42.57,26.18 42.58,26.18 arc90 42.62,26.21 v42.67,25.93 arc90 42.38,26.45 42.24,26.45 arc90 41.26,25.48 arc-90 39.62,23.84 25.4,23.84 arc90 22.52,20.95 22.52,20.32 arc-90 20.95,18.76 19.05,18.76 arc-90 18.12,19.68 arc90 16.51,21.3 9.53,21.3 arc90 8.93,20.7 8.93,19.61 arc-90 7.77,18.45 6.46,18.45 v6.25,18.29 5.79,18.5 PAD15.1
USBVDD  (via drill 0.38 pad 0.69)
  Top 0.305: v11.12,18.06 9.42,18.97 U10.6 8.2,19.91 7.47,20.62 7.09,21.01 v6.55,21.01 | J13.1 4.3,19.74 5.33,19.74 6.55,20.95 v6.55,21.01 | v6.55,21.01 6.38,21.18 FB1.1
  Top 0.356: J13.1
  Bottom 0.305: PAD13.1 v11.12,18.06
USBVSS  (via drill 0.38 pad 0.69)
  Top 0.305: U10.3 7.04,17.96 6.3,17.32 v6.3,16.31 | J13.5 5.56,17.12 v6.3,16.31 | v6.3,16.31 6.38,16.3 FB2.1
  Top 0.356: J13.5 | FB2.1 6.38,12.17 6.3,12.09 5.75,12.09 R44.2 5.69,12.03 5.69,11.38 5.59,11.28 3.15,11.28 3.14,11.29 C53.1
VCCAD
  Top 0.152: 100.99,20.95 100.99,21.44 101.19,21.64 101.19,22.17 100.81,22.55 100.81,23.87 U1.69
  Top 0.178: R4.2 97.18,20.95 97.18,20.32 98.4,20.32 | 98.4,20.32 98.42,20.3 R2.2 98.4,19.7 98.4,20.32 | 100.99,20.95 C19.1 100.47,20.92 100.43,20.88 100.43,20.37 100.38,20.32 98.4,20.32
  Top 0.254: R3.2 R4.2
VREFA+
  Top 0.152: U7.9 57.76,28.86 58.17,29.26 58.76,29.26 C48.1 58.78,29.89 62.24,29.89 63.42,31.06 64.26,31.06 U8.1 64.26,29.97 65.58,28.65 R40.2

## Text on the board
tNames: . | LIGHT SENSOR > | 20 | 11 | 60 | 51 | ERR | TMS570 / RM4x / 144 PGE LAUNCHPAD XL2 | +5V DC | 40 | 31 | 80 | 71 | XDS-110 EMULATOR | PORRST | +3V3 | KILL / OSC | RESET | . | USER LED A | GIOB_1 | SPI3NCS0/ | AD2EVT/ | XDS110 | <+5V | GIOB_2/ | Debug LEDS | QEP1I | USER SWITCH A | USER LED B | GIOB_2 | HET1_15 | +5V | 21 | 30 | LED7 LED8 / off off Not Ready / on off Ready To Connect / on on Connected / on blink Connected/Activity / off on Serious Error | 61 | 70 | SPI1NCS_4 | ECAP1 | +5V | USER SWITCH B | +3V3 | +3V3 | 1 | 10 | 50 | 41 | (C) 2014 Texas Instruments, Inc. | Pb | For evaluation only; not FCC approved for resale. | CURRLIM | Rev(B)
Document: NOTES: / ===== / 1) All dimensions in mils / 2) Build to IPC 6012 Class 2 / 3) FR4 Dielectric / 4) Finish Thickness 0.062" / 5) 1 Oz Copper Top/Bottom Layers / 6) 0.5 Oz Copper Inner Layers / 7) Lead-Free Solder Finish / 8) Red LPI Soldermask Both Sides / 9) White Silkscreen Both Sides / 10) ROHS / REACH Required / 11) UL94V-0 Required | Layer Stackup: / ========= / .SST Top Side Silkscreen - Positive / .SMT Top Side Soldermask - Positive / .TOP Top Copper (Layer 1) - Positive / .IN1 Inner Copper (Layer 2) - Positive / .IN2 Inner Copper (Layer 3) - Positive / .BOT Bottom Copper(Layer 4) - Positive / .SMB Bottom Soldermask - Positive / .SSB Bottom Silkscreen - Positive
DrillLegend: LAYER-STACK
DrillLegend_01-16: 01-16
210bmp: C:/Users/a0321811/Desktop/ce-mark.bmp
